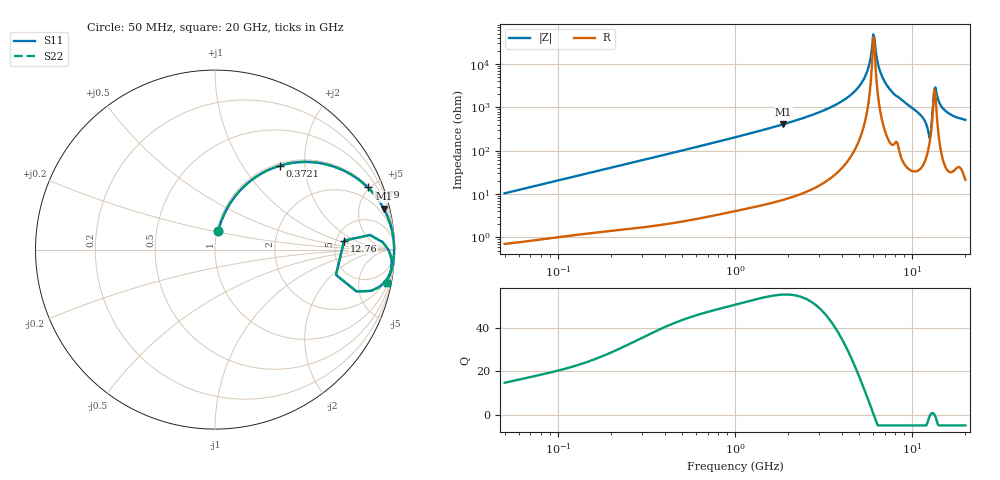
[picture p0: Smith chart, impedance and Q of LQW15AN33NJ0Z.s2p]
!Murata Part Number: LQW15AN33NJ0Z
!These Parameters are Measured in Series Mode Connection
!  o--[Z]--o
!Port1  Port2
!  o-------o
!Freq. Start=50[MHz] Stop=20[GHz], 401[Steps]
# Hz S RI R 50
!Freq.(Hz) S11(Real) S11(Imag) S21(Real) S21(Imag) S12(Real) S12(Imag) S22(Real) S22(Imag)
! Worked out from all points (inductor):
!   401 points, 50 MHz to 20 GHz, reference 50 ohm
!   read as one part in series: L = 33 nH near 51.52 MHz
!   highest Q = 55.3 at 1.876 GHz (marker M1), where L = 34.7 nH
!   self-resonance near 6.034 GHz
!   S11 on the Smith chart (normalised r, x): 50 MHz: 1.01, +0.21; 372.1 MHz: 1.04, +1.50; 1.179 GHz: 1.09, +4.86; 12.76 GHz: 5.91, +1.24; 20 GHz: 1, -10
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5e7  0.0175 0.1015  0.9825 -0.1015  0.9825 -0.1015  0.0175 0.1015
1.364002e8  0.0812 0.2527  0.9188 -0.2527  0.9188 -0.2527  0.0812 0.2527
3.721004e8  0.3637 0.4685  0.6363 -0.4685  0.6363 -0.4685  0.3637 0.4685
1e9  0.8021 0.3886  0.1979 -0.3886  0.1979 -0.3886  0.8021 0.3886
1.179116e9  0.8506 0.347  0.1494 -0.347  0.1494 -0.347  0.8506 0.347
1.875929e9  0.94 0.2287  0.06 -0.2287  0.06 -0.2287  0.94 0.2287
2.728004e9  0.9756 0.145  0.0244 -0.145  0.0244 -0.145  0.9756 0.145
3.908127e9  0.992 0.0762  0.00795 -0.0762  0.00795 -0.0762  0.992 0.0762
4.89267e9  0.9968 0.0369  0.00323 -0.0369  0.00323 -0.0369  0.9968 0.0369
5.515528e9  0.9979 0.0165  0.00208 -0.0165  0.00208 -0.0165  0.9979 0.0165
6.034176e9  0.9982 0.00102  0.0018 -0.00102  0.0018 -0.00102  0.9982 0.00102
6.217679e9  0.9982 -0.00417  0.00183 0.00417  0.00183 0.00417  0.9982 -0.00417
6.701223e9  0.9978 -0.0174  0.00217 0.0174  0.00217 0.0174  0.9978 -0.0174
7.442007e9  0.9964 -0.0367  0.00356 0.0367  0.00356 0.0367  0.9964 -0.0367
1.131968e10  0.9656 -0.1522  0.0344 0.1522  0.0344 0.1522  0.9656 -0.1522
1.238412e10  0.789 -0.2336  0.211 0.2336  0.211 0.2336  0.789 -0.2336
1.276073e10  0.7197 0.0503  0.2803 -0.0503  0.2803 -0.0503  0.7197 0.0503
1.334722e10  0.9627 0.00459  0.0373 -0.00459  0.0373 -0.00459  0.9627 0.00459
1.375312e10  0.9806 -0.0429  0.0194 0.0429  0.0194 0.0429  0.9806 -0.0429
1.460232e10  0.9837 -0.0908  0.0163 0.0908  0.0163 0.0908  0.9837 -0.0908
1.550395e10  0.9796 -0.1188  0.0204 0.1188  0.0204 0.1188  0.9796 -0.1188
2e10  0.9564 -0.1844  0.0436 0.1844  0.0436 0.1844  0.9564 -0.1844
